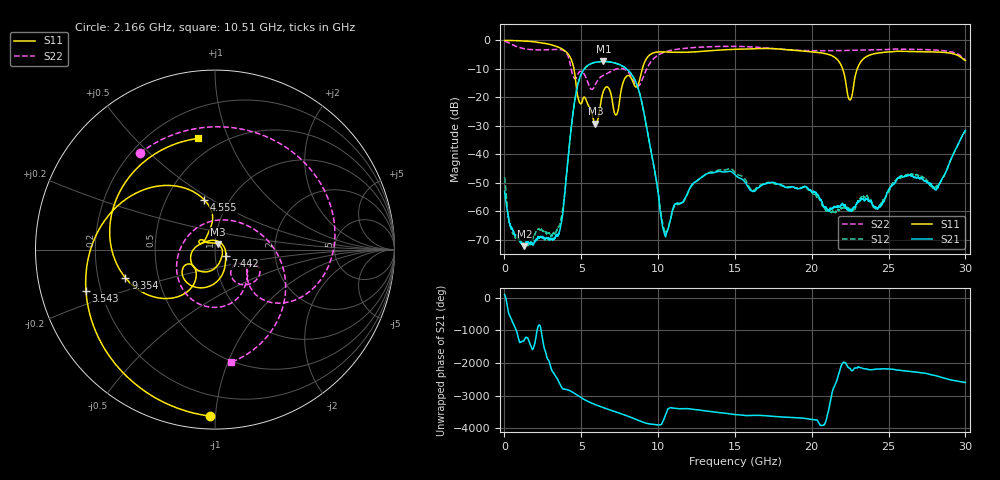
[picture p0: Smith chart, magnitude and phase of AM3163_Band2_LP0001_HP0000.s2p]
!Agilent Technologies,E8364B,MY43040894,A.07.50.67
!Agilent E8364B: A.07.50.67
!Date: Thursday, August 20, 2020 12:04:29
!Correction: S11(Full 2 Port(1,2))
!S21(Full 2 Port(1,2))
!S12(Full 2 Port(1,2))
!S22(Full 2 Port(1,2))
!S2P File: Measurements: S11, S21, S12, S22:
# Hz S  dB  R 50
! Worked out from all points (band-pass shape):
!   3201 points, 10 MHz to 30 GHz, reference 50 ohm
!   highest |S21| = -7.39 dB at 6.439 GHz (marker M1); lowest = -72.3 dB at 1.303 GHz (marker M2)
!   |S21| within 3 dB of the highest: 5.149 GHz to 8.025 GHz (2.876 GHz wide, 43.7 % of centre)
!   lowest |S11| = -29.3 dB at 5.924 GHz (marker M3), VSWR 1.07, Z = 51.4 + j3.2 ohm
!   |S11| at or under -10 dB: 4.523 GHz to 8.973 GHz (4.449 GHz wide, 65.9 % of centre); 22.01 GHz to 22.96 GHz (950.7 MHz wide, 4.23 % of centre)
!   |S22| runs from -17.2 to -0.3 dB; largest |S21 - S12| = 0.0033
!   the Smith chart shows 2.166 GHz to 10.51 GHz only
!   S11 on the Smith chart (normalised r, x): 2.166 GHz: 0.07, -0.97; 3.543 GHz: 0.14, -0.15; 4.555 GHz: 0.77, +0.46; 7.442 GHz: 1.13, -0.07; 9.354 GHz: 0.32, -0.14; 10.51 GHz: 0.38, +0.78
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1e7  -0.02 -2.8  -53.09 94.7  -48.06 134.2  -0.29 -12.0
5.441969e8  -0.05 -22.4  -66.92 -49.6  -67.93 1.1  -1.60 -85.6
1.303319e9  -0.20 -54.2  -72.32 155.1  -72.30 42.3  -2.93 -166.5
2.165531e9  -0.65 -91.7  -68.92 150.8  -66.50 -0.5  -3.34 127.9
3.543197e9  -2.44 -162.3  -67.90 -68.6  -65.54 170.1  -3.18 30.3
4.555359e9  -10.96 102.1  -21.87 -53.7  -21.90 -53.9  -13.35 -33.3
5.014581e9  -22.18 149.7  -11.66 164.4  -11.66 164.2  -10.93 -37.7
5.923653e9  -29.25 64.4  -7.68 -41.5  -7.69 -41.6  -15.47 -28.5
6.439106e9  -17.91 -106.5  -7.39 -131.6  -7.39 -131.8  -12.29 -42.8
7.441897e9  -23.23 -28.7  -8.39 66.3  -8.44 66.3  -9.87 -84.8
8.210391e9  -12.88 -143.8  -11.48 -65.2  -11.48 -65.0  -12.30 -151.5
9.353759e9  -5.62 -162.6  -33.60 98.0  -33.43 97.6  -9.01 -5.6
1.000979e10  -4.06 137.8  -53.68 56.2  -53.65 57.5  -5.14 -55.8
1.05065e10  -4.06 98.8  -68.70 36.0  -67.28 153.7  -3.95 -82.0
1.213721e10  -4.11 -11.4  -51.27 -172.7  -51.55 -169.1  -2.58 -143.4
1.5005e10  -3.11 -144.3  -47.15 17.2  -46.37 17.4  -2.10 124.8
1.767598e10  -2.93 93.7  -50.25 -45.4  -50.57 -49.5  -2.97 27.0
2.000958e10  -4.02 -31.7  -53.27 -132.4  -53.18 -122.7  -3.60 -53.3
2.248376e10  -20.92 -104.3  -59.89 -5.8  -59.59 -112.2  -3.50 -122.7
2.500479e10  -4.07 -151.7  -52.34 -25.1  -53.18 -26.5  -3.18 175.8
2.811625e10  -4.08 110.5  -52.28 121.4  -51.08 126.3  -3.41 93.2
3e10  -7.08 39.5  -31.63 -80.2  -32.02 -79.0  -6.82 36.0
